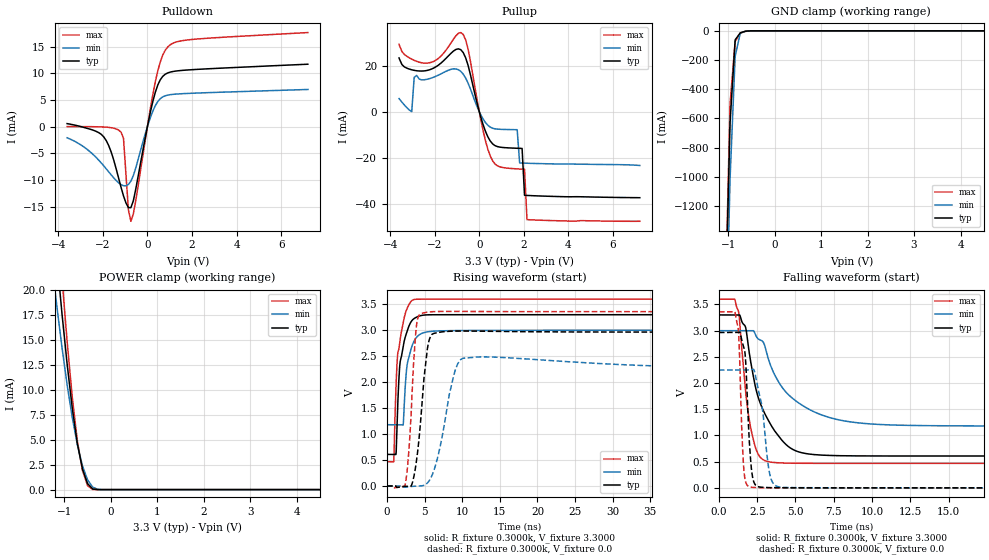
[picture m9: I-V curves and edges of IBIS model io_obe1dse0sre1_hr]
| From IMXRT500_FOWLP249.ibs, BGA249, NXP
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[Model] io_obe1dse0sre1_hr
|   Model io_obe1dse0sre1_hr
| Library cells for typ/min/max conditions are connected as defined below:
|  pad - External Pad
|  ipp_do - Core Input
|  ipp_obe - Output Buffer Enable
|  REFH3V3 - vdd1v8
|  REFL3V3 - vdd1v8
|  gnde - gnde
|  ipp_ina235_3v - NC
|  ipp_ina40_3v - NC
|  ipp_ina_mux - NC
|  ipp_ind - NC
|  ipp_ind_1p8v - NC
|  ipp_ind_3v - NC
|  ipp_sre - vdd
|  vdd - vdd
|  vdd1v8 - vdd1v8
|  vdda - vdde3v3
|  vdde3v3 - vdde3v3
| All other pins connected to ground
Model_type I/O
Polarity   Non-Inverting
Enable   Active-High
Vinl =   0.9900V
Vinh =   2.3100V
Vmeas =  1.6500V
Cref =   25.0000pF
Rref =   0.5000k
Vref =   0.0V
C_comp   1.8292pF   1.7593pF   1.9120pF
[Temperature Range]   25.0000   0.1250k   -40.0000
[Voltage Range]   3.3000V   3.0000V   3.6000V
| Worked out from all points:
|   slope of the pulldown table from 0 to 0.495 V, typ, clamps not added: 61.4 ohm
|   slope of the pullup table from 0 to 0.495 V, typ, clamps not added: 38.6 ohm
|   GND clamp passes 1 mA (typ) near -0.55 V on its own axis
|   POWER clamp passes 1 mA (typ) near -0.53 V on its own axis
|   rising waveform, R_fixture 0.3000k, V_fixture 3.3000: 20-80 % time 919ps typ, 907ps min, 901ps max; typ from 0.608 V to 3.3 V
|   rising waveform, R_fixture 0.3000k, V_fixture 0.0: 20-80 % time 1.12ns typ, 1.79ns min, 780ps max; typ from 0 V to 2.96 V
|   falling waveform, R_fixture 0.3000k, V_fixture 3.3000: 20-80 % time 1.62ns typ, 2.55ns min, 705ps max; typ from 3.3 V to 0.608 V
|   falling waveform, R_fixture 0.3000k, V_fixture 0.0: 20-80 % time 298ps typ, 584ps min, 230ps max; typ from 2.96 V to 0 V
[Pulldown]
|Voltage   I(typ)   I(min)   I(max)
-3.6V     580uA      -2.07mA    30uA
-1.95V    -1.94mA    -7.35mA    -60uA
-1.62V    -4.77mA    -9.02mA    -190uA
-1.18V    -11.35mA   -10.84mA   -1.013mA
-1.07V    -12.94mA   -11.04mA   -2.193mA
-850mV    -15.13mA   -10.79mA   -15.56mA
-740mV    -15.14mA   -10.18mA   -17.69mA
-520mV    -11.65mA   -7.709mA   -13.83mA
360mV     6.495mA    3.971mA    8.469mA
580mV     8.787mA    5.251mA    12.13mA
910mV     10.06mA    5.911mA    14.9mA
7.2V      11.7mA     6.967mA    17.61mA
[Pullup]
|Voltage   I(typ)   I(min)   I(max)
-3.6V     23.39mA    5.712mA    29.31mA
-3.03V    18.24mA    68.6uA     22.87mA
-2.92V    17.99mA    14.95mA    22.35mA
-2.26V    18.16mA    14.31mA    21.23mA
-720mV    25.7mA     16.34mA    33.57mA
490mV     -12.7mA    -6.677mA   -19.19mA
1.7V      -15.88mA   -7.809mA   -24.84mA
1.81V     -15.91mA   -22.26mA   -24.9mA
1.92V     -15.95mA   -22.31mA   -24.96mA
2.03V     -36.32mA   -22.35mA   -25.02mA
2.14V     -36.38mA   -22.39mA   -46.91mA
7.2V      -37.37mA   -23.36mA   -47.62mA
[GND_clamp]
|Voltage   I(typ)   I(min)   I(max)
-3.6V     -46.64A    -46.27A    -48.09A
-1.07V    -2.038A    -2.424A    -1.965A
-960mV    -629.9mA   -1.012A    -499.2mA
-850mV    -61.62mA   -174.1mA   -72.03mA
-740mV    -13.6mA    -15.66mA   -16.3mA
-630mV    -2.66mA    -3.244mA   -3.912mA
-410mV    -9.358uA   -49.22uA   -3.515uA
7.2V      0A         0A         0A
[POWER_clamp]
|Voltage   I(typ)   I(min)   I(max)
-3.6V     129.4mA    109.3mA    143.3mA
-1.27V    28.99mA    22.71mA    35.27mA
-1.16V    23.09mA    18.31mA    28mA
-1.05V    17.57mA    14.21mA    21.12mA
-940mV    12.56mA    10.49mA    14.82mA
-830mV    8.174mA    7.224mA    9.263mA
-720mV    4.592mA    4.483mA    4.857mA
-610mV    2.058mA    2.37mA     1.909mA
-500mV    597.2uA    970.5uA    391.6uA
-390mV    63.24uA    245.6uA    14.23uA
-170mV    54.62nA    1.775uA    12.62nA
7.2V      0A         0A         0A
[Ramp]
| variable   typ   min   max
dV/dt_r  0.6651/1.4796n   0.6687/3.9117n   0.7549/0.9718n
dV/dt_f  0.3253/1.9068n   0.1910/2.4912n   0.4971/1.1025n
R_load = 50.0000
[Rising Waveform]
R_fixture= 0.3000k
V_fixture= 3.3000
V_fixture_min= 3.0000
V_fixture_max= 3.6000
|time   V(typ)   V(min)   V(max)
0s        607.6mV    1.18V      467.4mV
902.6ps   607.6mV    1.18V      472.5mV
1.207ns   623.9mV    1.18V      1.946V
1.357ns   1.286V     1.18V      2.423V
1.657ns   2.241V     1.18V      2.725V
1.897ns   2.478V     1.179V     2.956V
2.168ns   2.708V     1.201V     3.157V
2.704ns   2.99V      2.358V     3.429V
3.887ns   3.25V      2.856V     3.598V
500ns     3.3V       3V         3.6V
[Rising Waveform]
R_fixture= 0.3000k
V_fixture= 0.0
V_fixture_min= 0.0
V_fixture_max= 0.0
|time   V(typ)   V(min)   V(max)
0s        327.7nV    1.778uV    1.402uV
2.392ns   -10.49mV   -22.35mV   7.678mV
2.885ns   -6.613mV   -13.31mV   629.1mV
3.361ns   54.48mV    -8.59mV    1.859V
4.075ns   659.9mV    -3.5mV     3.222V
5.299ns   2.57V      45.77mV    3.348V
6.167ns   2.936V     269.9mV    3.359V
9.369ns   2.984V     2.344V     3.363V
12.35ns   2.982V     2.486V     3.361V
500ns     2.965V     2.248V     3.358V
[Falling Waveform]
R_fixture= 0.3000k
V_fixture= 3.3000
V_fixture_min= 3.0000
V_fixture_max= 3.6000
|time   V(typ)   V(min)   V(max)
0s        3.3V       3V         3.6V
1.031ns   3.3V       3V         3.601V
1.279ns   3.299V     3V         3.368V
1.86ns    2.837V     3V         1.541V
2.488ns   1.806V     2.868V     689.8mV
3.353ns   1.223V     2.353V     493.1mV
4.437ns   812.2mV    1.809V     472mV
7.9ns     613.7mV    1.293V     467.4mV
15.4ns    607.7mV    1.183V     467.4mV
500ns     607.6mV    1.18V      467.4mV
[Falling Waveform]
R_fixture= 0.3000k
V_fixture= 0.0
V_fixture_min= 0.0
V_fixture_max= 0.0
|time   V(typ)   V(min)   V(max)
0s        2.965V     2.248V     3.358V
1.248ns   2.965V     2.248V     3.071V
1.335ns   2.971V     2.248V     2.641V
1.523ns   2.783V     2.248V     900mV
1.659ns   2.654V     2.248V     257.2mV
2.118ns   378.5mV    2.252V     11.61mV
2.595ns   20.02mV    1.841V     3.722mV
3.409ns   4.195mV    167.2mV    977.3uV
4.891ns   1.049mV    4.783mV    117.9uV
500ns     1.532uV    3.285uV    3.235uV
